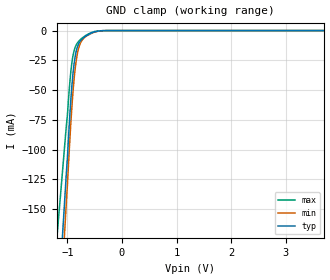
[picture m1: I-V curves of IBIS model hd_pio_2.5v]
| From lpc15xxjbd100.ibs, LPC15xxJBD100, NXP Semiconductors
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[Model] hd_pio_2.5v
Model_type Input
Vinl = 990.000mV
Vinh = 2.31000V
C_comp 598.000fF 598.000fF 598.000fF
| variable typ   min   max
[Voltage Range] 2.50000V 2.25000V 2.75000V
[POWER Clamp Reference] 2.50000V 2.25000V 2.75000V
[GND Clamp Reference] 0.00000V 0.00000V 0.00000V
[Temperature Range]   25   85   -40
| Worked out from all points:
|   GND clamp passes 1 mA (typ) near -0.49 V on its own axis
[GND Clamp]
-2.5V     -1.219A    -1.334A    -886mA
-1.02V    -120mA     -144.3mA   -80.04mA
-1V       -106.5mA   -129.2mA   -70.92mA
-960mV    -73.92mA   -95.1mA    -45.49mA
-920mV    -47.27mA   -65.11mA   -27.49mA
-880mV    -28.66mA   -41.65mA   -17.27mA
-840mV    -17.58mA   -25.47mA   -12.14mA
-800mV    -11.7mA    -15.74mA   -9.357mA
-760mV    -8.541mA   -10.37mA   -7.463mA
-580mV    -2.501mA   -2.825mA   -2.036mA
-280mV    0A         0A         0A
5V        0A         0A         0A
[POWER Clamp]
-2.5V     0A         0A         0A
5V        0A         0A         0A
